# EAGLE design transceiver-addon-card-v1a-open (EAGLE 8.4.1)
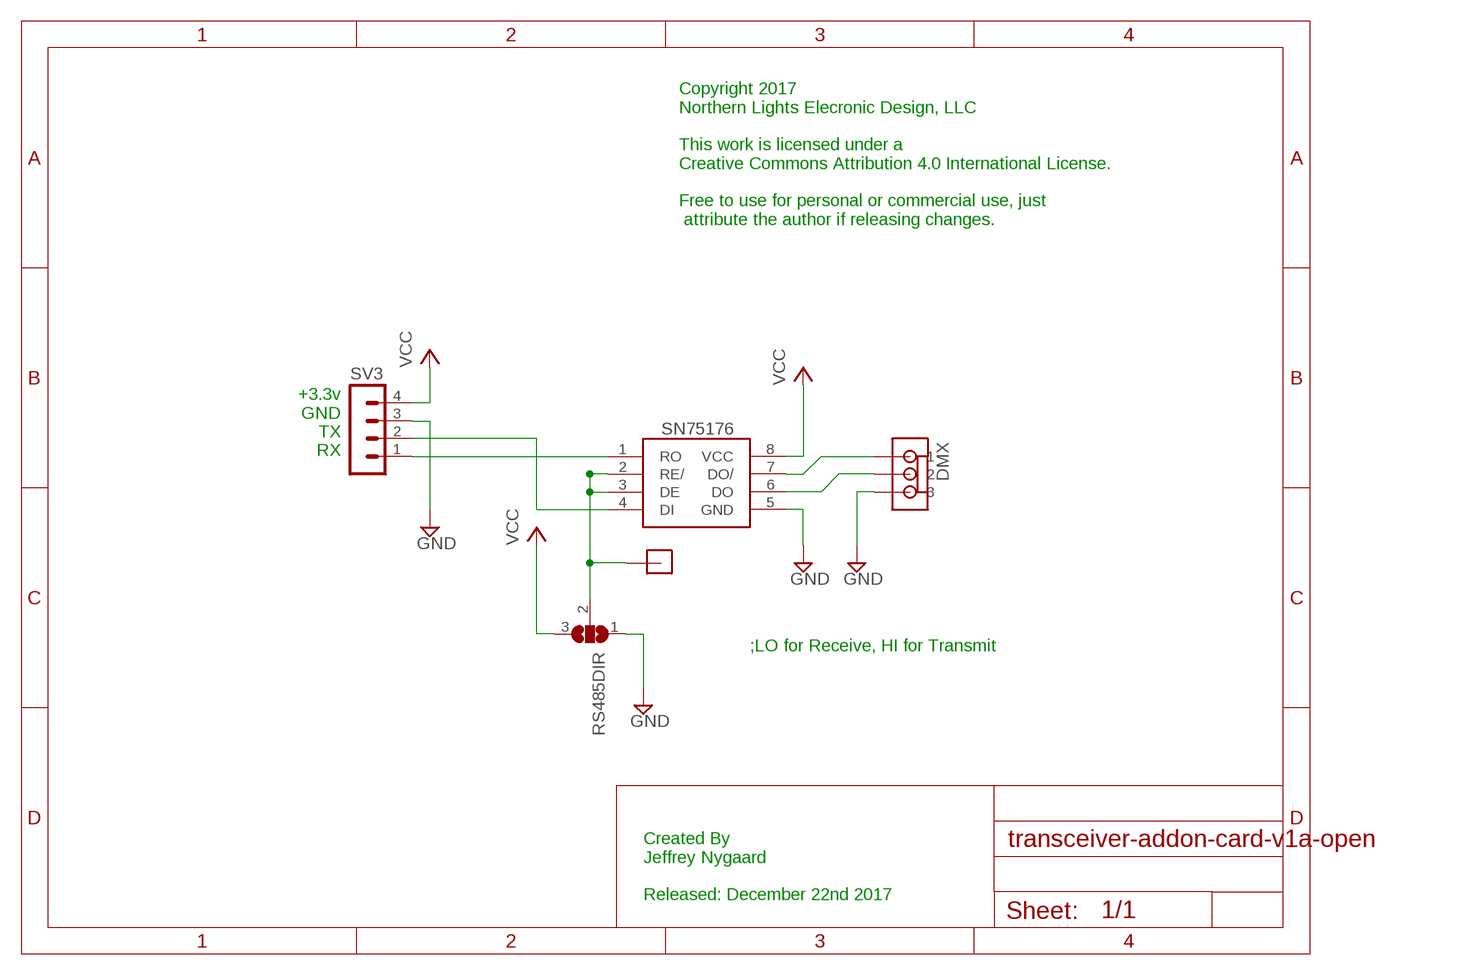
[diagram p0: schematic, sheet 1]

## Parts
DIR  JUMPER  [JUMPER]
DMX  MOLEXKK3  [MOLEXKK3]
RS485DIR  SJ2W  [SJ_2]
SN75176  SN75176SMD  [SOIC-8]
SV3  MA04-1  [MA04-1]

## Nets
GND: DMX.3 RS485DIR.1 SN75176.5(GND) SV3.3
N$1: DMX.2 SN75176.6(DO)
N$2: DMX.1 SN75176.7(DO/)
N$11: SN75176.1(RO) SV3.1
N$12: DIR.2(J1) RS485DIR.2 SN75176.2(RE/) SN75176.3(DE)
N$16: SN75176.4(DI) SV3.2
VCC: RS485DIR.3 SN75176.8(VCC) SV3.4

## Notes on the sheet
- Copyright 2017
  Northern Lights Elecronic Design, LLC
  
  This work is licensed under a 
  Creative Commons Attribution 4.0 International License.
  
  Free to use for personal or commercial use, just
   attribute the author if releasing changes.
- +3.3v
  GND
  TX
  RX
- ;LO for Receive, HI for Transmit
- Created By
  Jeffrey Nygaard
  
  Released: December 22nd 2017

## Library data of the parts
DIR = ChromationSystems-1:JUMPER
DMX = ChromationSystems-1:MOLEXKK3
RS485DIR = jumper:SJ2W: SMD solder JUMPER
SN75176 = ChromationSystems-2:SN75176
SV3 = ChromationSystems-2:MA04-1: PIN HEADER; OC_FARNELL: unknown; OC_NEWARK: unknown

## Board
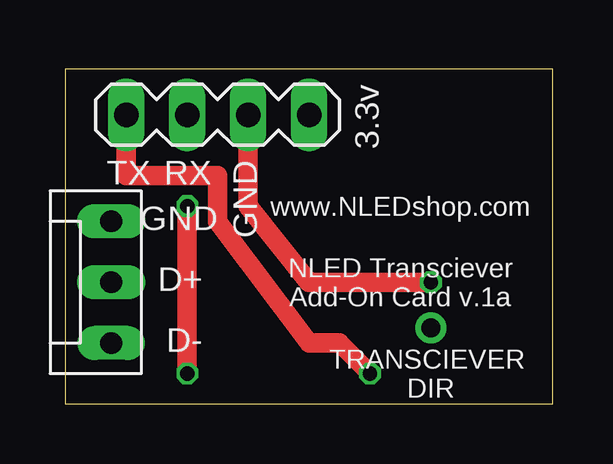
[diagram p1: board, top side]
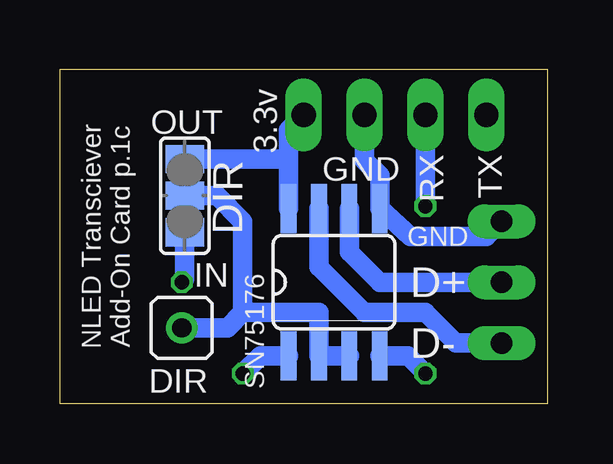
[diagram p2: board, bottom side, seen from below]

Size 20.32 x 13.97 mm. Coordinates in mm from the lower left corner, seen from the top.
Outline: 0,0 20.32,0 20.32,13.97 0,13.97 0,0
Copper layers (1*16): Top 0.035mm / dielectric 1.5mm / Bottom 0.035mm
Design rules "SeeedStudio_2layer_DRU_no_angle_20140221": minimum track width 6mil, minimum drill 12mil, track to track 6mil, track to pad 6mil, pad to pad 6mil, via to via 6mil, smd to smd 0mil, copper to edge 10mil, drill to drill 10mil, minimum pad ring 10mil, minimum via ring 6mil, stop-mask expansion 2mil, vias tented up to drill 100mil, thermal gap 10mil

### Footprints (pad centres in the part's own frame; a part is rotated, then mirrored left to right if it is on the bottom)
JUMPER = drill 0.8: 2 0,0
MOLEXKK3 = drill 0.9 long: 1 -2.54,0 | drill 0.9 pad 1.422 long: 2 0,0; 3 2.54,0
SJ_2 = smd 1.168 x 1.6: 1 -1.524,0; 2 0,0; 3 1.524,0
SOIC-8 = smd 0.66 x 2.032: 1 -1.905,-3.073; 2 -0.635,-3.073; 3 0.635,-3.073; 4 1.905,-3.073; 5 1.905,3.073; 6 0.635,3.073; 7 -0.635,3.073; 8 -1.905,3.073
MA04-1 = drill 1.016 long: 1 -3.81,0; 2 -1.27,0; 3 1.27,0; 4 3.81,0

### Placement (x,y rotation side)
DIR  15.24,3.17 0 bottom
DMX  1.91,5.08 90 top
RS485DIR  15.11,8.69 90 bottom
SN75176  8.89,5.08 0 bottom
SV3  6.35,12.06 0 top

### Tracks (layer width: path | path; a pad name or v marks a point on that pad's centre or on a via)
GND  (via drill 0.6)
  Top 0.813: v15.24,5.08 10.16,5.08 7.62,8.26 SV3.3
  Bottom 0.813: SV3.3 7.62,10.16 6.99,9.53 SN75176.5 5.71,6.99 2.54,6.99 DMX.3 | RS485DIR.1 15.11,5.21 v15.24,5.08
N$1
  Bottom 0.813: SN75176.6 8.26,6.35 6.99,5.08 DMX.2
N$2
  Bottom 0.813: DMX.1 3.81,2.54 5.08,3.81 7.62,3.81 9.53,5.71 SN75176.7
N$11  (via drill 0.6)
  Top 0.813: SV3.1 2.54,9.53 6.35,9.53 6.35,7.62 10.16,2.54 11.43,2.54 v12.7,1.27
  Bottom 0.813: SN75176.1 11.96,2.01 v12.7,1.27
N$12
  Bottom 0.813: SN75176.3 SN75176.2 9.53,3.81 12.7,3.81 | RS485DIR.2 13.77,8.69 12.7,7.62 12.7,3.81 | 12.7,3.81 13.34,3.17 DIR.2
N$16  (via drill 0.6)
  Top 0.813: v5.08,8.26 v5.08,1.27
  Bottom 0.813: SN75176.4 5.82,2.01 v5.08,1.27 | SV3.2 v5.08,8.26
VCC
  Bottom 0.813: SN75176.8 10.79,10.16 | 10.79,10.16 10.79,11.43 SV3.4 | RS485DIR.3 10.85,10.21 10.79,10.16

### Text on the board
tNames: 3.3v | TX | RX | GND | GND | www.NLEDshop.com | D+ | NLED Transciever / Add-On Card v.1a | D- | TRANSCIEVER / DIR
bNames: 3.3v | OUT | TX | RX | GND | GND | NLED Transciever / Add-On Card p.1c | IN | D+ | D- | DIR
